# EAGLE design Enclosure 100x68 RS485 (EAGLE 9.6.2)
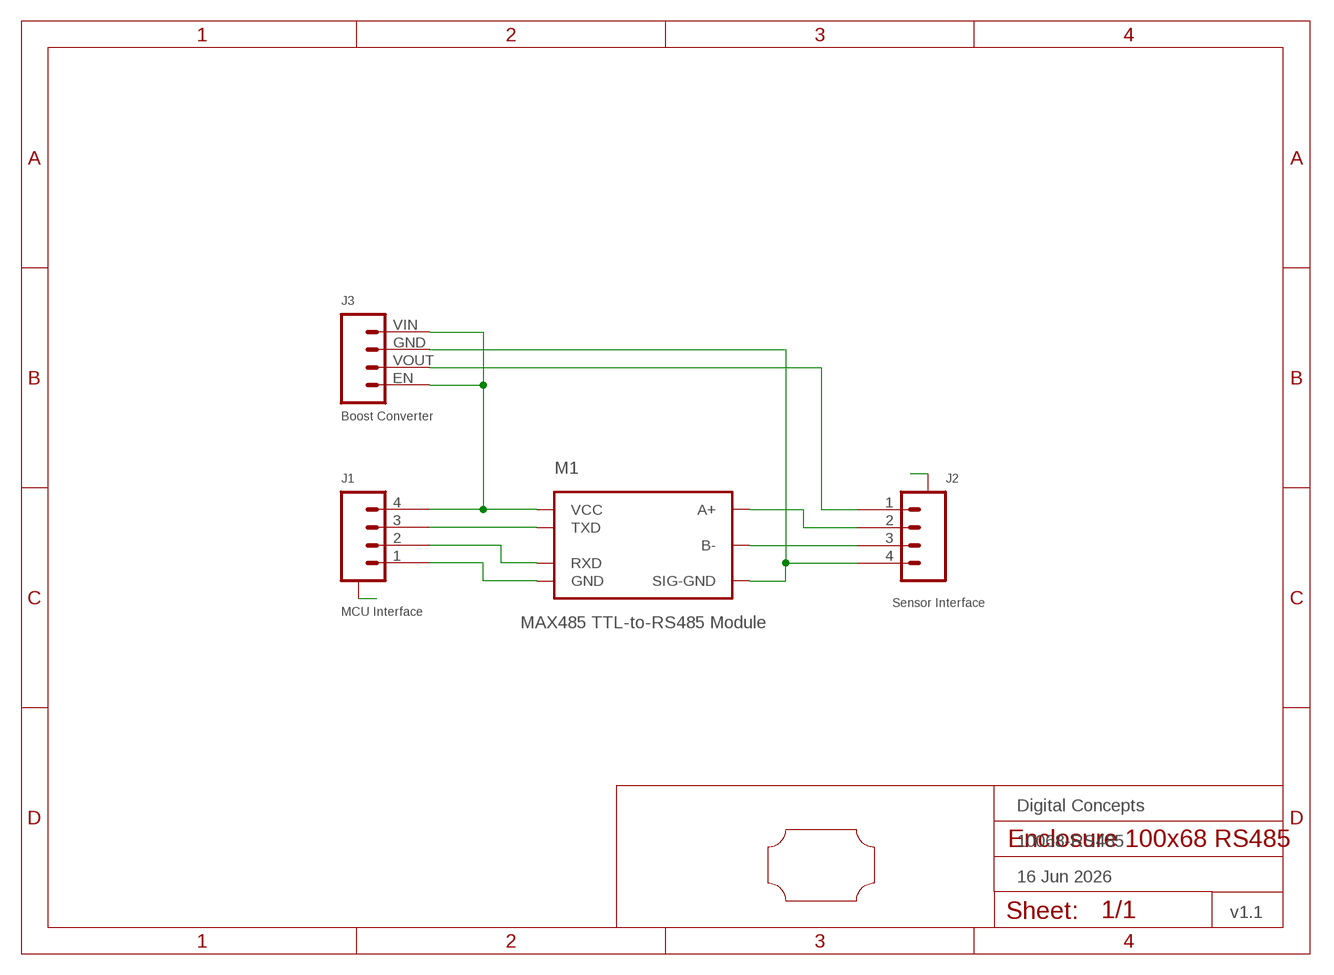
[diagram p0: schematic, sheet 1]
FRAME1 (FRAME_A5L-LOC): DATE: 16 Jun 2026; OWNER: Digital Concepts; TITLE: 10068-RS485; VERSION: v1.1

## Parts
J1  MCU Interface  JST-SH1.0-4-SMD-HORIZONTAL  [JST-SH1.0-4-SMD-HORIZONTAL]
J2  Sensor Interface  JST-SH1.0-4-SMD-HORIZONTAL  [JST-SH1.0-4-SMD-HORIZONTAL]
J3  Boost Converter  HEADER-1X4-BOOST  [CONN_04-BOOST]
M1  MAX485 TTL-to-RS485 Module  MAX485-MODULE  [MAX485-MODULE]
U$1  PROTO-34X22-RS485  [PROTO-34X22-RS485]

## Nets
A1: J2.A@1(A) J2.A@4(A)
A2: J1.A@1(A) J1.A@4(A)
A+: J2.2 M1.A+
B-: J2.3 M1.B-
GND: J1.1 M1.GND
RXD: J1.2 M1.RXD
SIG-GND: J2.4 J3.GND M1.SIG-GND
TXD: J1.3 M1.TXD
VCC: J1.4 J3.EN J3.VIN M1.VCC
VDD: J2.1 J3.VOUT

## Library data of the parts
J1 J2 = digitalconcepts:JST-SH1.0-4-SMD-HORIZONTAL: JST SH1.0 4P SMD horizontal connector
J3 = digitalconcepts:HEADER-1X4-BOOST: Boost Converter Module 4-Pin Header
M1 = digitalconcepts:MAX485-MODULE: MAX485 TTL-to-RS485 Adaptor Module
U$1 = digitalconcepts:PROTO-34X22-RS485: 34 x 22 Prototyping board, with cut-outs, to fit an 100 x 68 enclosure

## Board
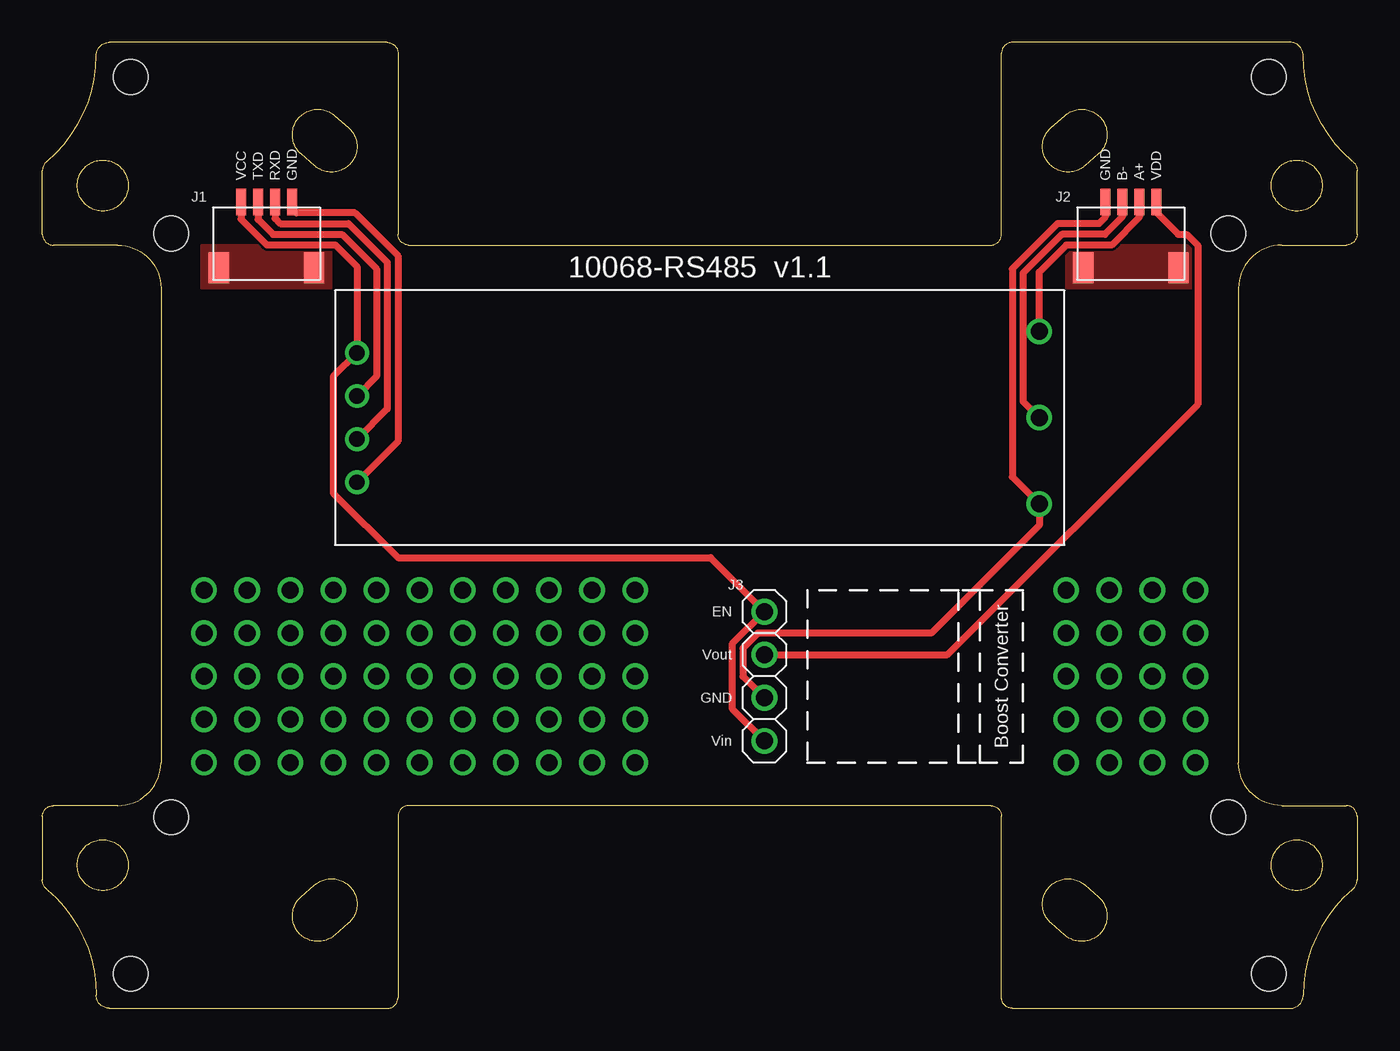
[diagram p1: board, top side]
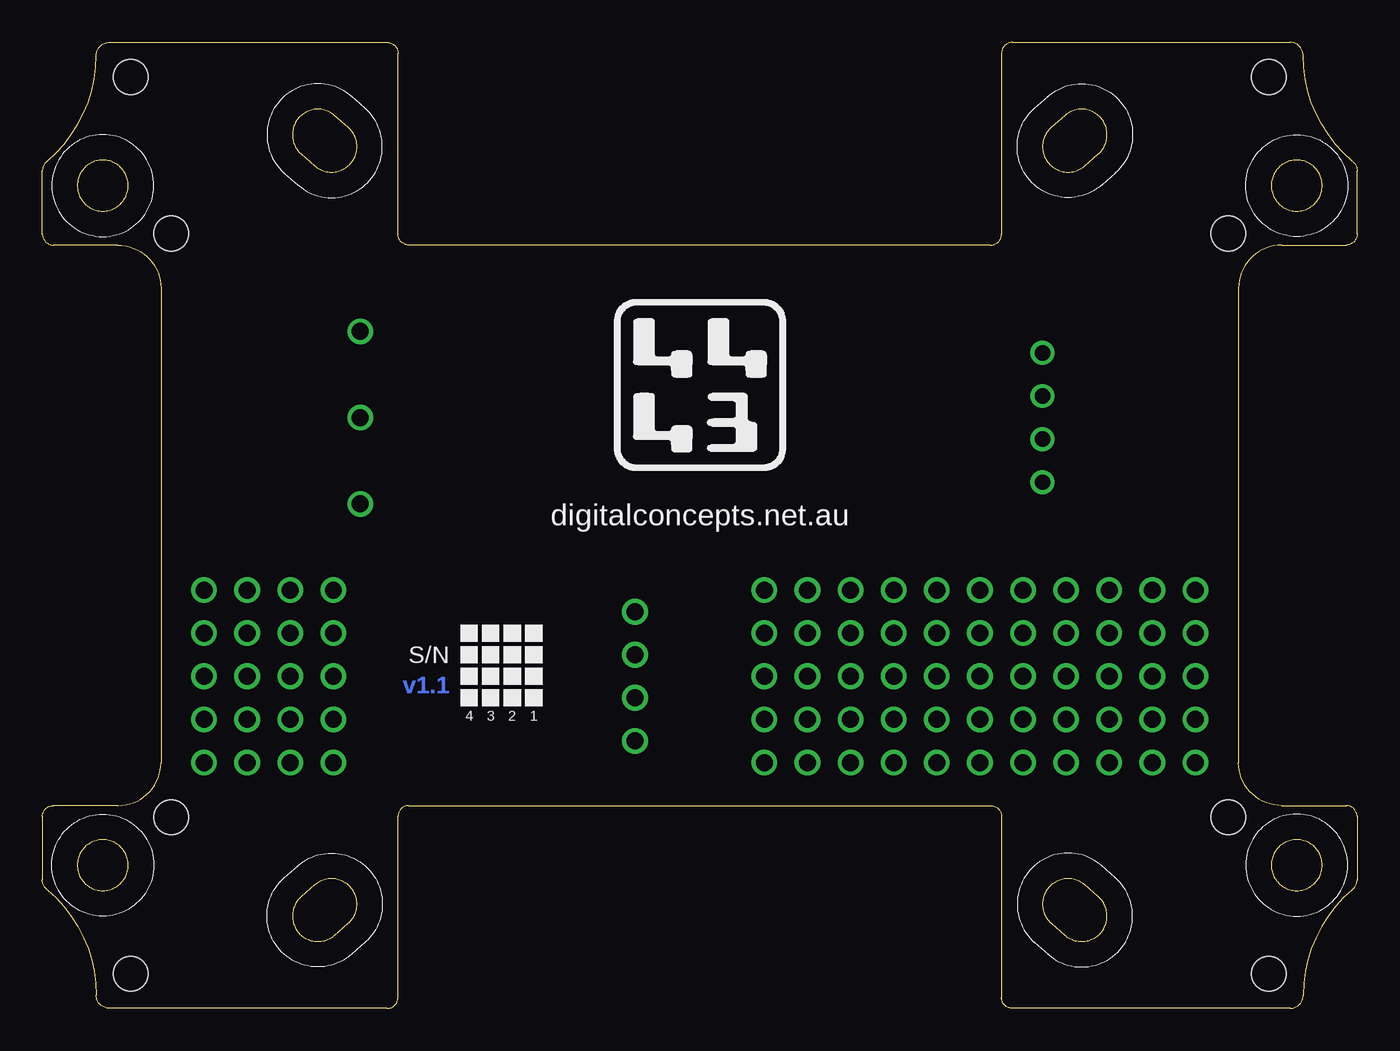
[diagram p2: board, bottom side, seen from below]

Size 77.47 x 56.9 mm. Coordinates in mm from the lower left corner, seen from the top.
Copper layers (1*16): Top 0.035mm / dielectric 1.5mm / Bottom 0.035mm
Design rules "default *": minimum track width 6mil, minimum drill 0.35mm, track to track 6mil, track to pad 6mil, pad to pad 6mil, via to via 6mil, smd to smd 6mil, copper to edge 6mil, drill to drill 6mil, minimum pad ring 10mil, minimum via ring 8mil, stop-mask expansion 4mil, vias tented up to drill 0mil, thermal gap 10mil

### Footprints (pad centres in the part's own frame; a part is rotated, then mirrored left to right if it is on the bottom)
JST-SH1.0-4-SMD-HORIZONTAL = smd 0.6 x 1.55: 1 1.5,2.54; 2 0.5,2.54; 3 -0.5,2.54; 4 -1.5,2.54 | smd 1.2 x 1.8: A@1 2.8,-1.335; A@4 -2.8,-1.335
CONN_04-BOOST = drill 1 pad 1.524: EN 0,0; GND 5.08,0; VIN 7.62,0; VOUT 2.54,0
MAX485-MODULE = drill 1: A+ 20,5.08; B- 20,0; SIG-GND 20,-5.08 | drill 0.9: GND -20.2,-3.81; RXD -20.2,-1.27; TXD -20.2,1.27; VCC -20.2,3.81
PROTO-34X22-RS485 = drill 1: P06-06 -29.21,-13.97; P06-07 -29.21,-11.43; P06-08 -29.21,-8.89; P06-09 -29.21,-6.35; P06-10 -29.21,-3.81; P07-06 -26.67,-13.97; P07-07 -26.67,-11.43; P07-08 -26.67,-8.89; P07-09 -26.67,-6.35; P07-10 -26.67,-3.81; P08-06 -24.13,-13.97; P08-07 -24.13,-11.43; P08-08 -24.13,-8.89; P08-09 -24.13,-6.35; P08-10 -24.13,-3.81; P09-06 -21.59,-13.97; P09-07 -21.59,-11.43; P09-08 -21.59,-8.89; P09-09 -21.59,-6.35; P09-10 -21.59,-3.81; P10-06 -19.05,-13.97; P10-07 -19.05,-11.43; P10-08 -19.05,-8.89; P10-09 -19.05,-6.35; P10-10 -19.05,-3.81; P11-06 -16.51,-13.97; P11-07 -16.51,-11.43; P11-08 -16.51,-8.89; P11-09 -16.51,-6.35; P11-10 -16.51,-3.81; P12-06 -13.97,-13.97; P12-07 -13.97,-11.43; P12-08 -13.97,-8.89; P12-09 -13.97,-6.35; P12-10 -13.97,-3.81; P13-06 -11.43,-13.97; P13-07 -11.43,-11.43; P13-08 -11.43,-8.89; P13-09 -11.43,-6.35; P13-10 -11.43,-3.81; P14-06 -8.89,-13.97; P14-07 -8.89,-11.43; P14-08 -8.89,-8.89; P14-09 -8.89,-6.35; P14-10 -8.89,-3.81; P15-06 -6.35,-13.97; P15-07 -6.35,-11.43; P15-08 -6.35,-8.89; P15-09 -6.35,-6.35; P15-10 -6.35,-3.81; P16-06 -3.81,-13.97; P16-07 -3.81,-11.43; P16-08 -3.81,-8.89; P16-09 -3.81,-6.35; P16-10 -3.81,-3.81; P26-06 21.59,-13.97; P26-07 21.59,-11.43; P26-08 21.59,-8.89; P26-09 21.59,-6.35; P26-10 21.59,-3.81; P27-06 24.13,-13.97; P27-07 24.13,-11.43; P27-08 24.13,-8.89; P27-09 24.13,-6.35; P27-10 24.13,-3.81; P28-06 26.67,-13.97; P28-07 26.67,-11.43; P28-08 26.67,-8.89; P28-09 26.67,-6.35; P28-10 26.67,-3.81; P29-06 29.21,-13.97; P29-07 29.21,-11.43; P29-08 29.21,-8.89; P29-09 29.21,-6.35; P29-10 29.21,-3.81 | hole 2.032: -33.528,26.416; 33.528,26.416; 33.528,-26.416; -33.528,-26.416; -31.14,17.196; 31.14,17.196; -31.14,-17.196; 31.14,-17.196

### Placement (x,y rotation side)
J1  13.21,44.96 0 top
J2  64.14,44.96 0 top
J3  42.55,23.37 270 top
M1  38.73,34.8 0 top
U$1  38.73,28.45 0 top

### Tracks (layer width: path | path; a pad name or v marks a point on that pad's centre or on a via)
A1
  pour Top (no thermals): 60.33,42.42 67.94,42.42 67.94,44.96 60.33,44.96
A2
  pour Top (no thermals): 9.4,44.96 17.02,44.96 17.02,42.42 9.4,42.42
A+
  Top 0.406: J2.2 64.64,46.59 63.01,44.96 60.33,44.96 58.73,43.37 M1.A+
B-
  Top 0.406: M1.B- 57.78,35.75 57.78,43.31 60.07,45.59 62.61,45.59 63.64,46.62 J2.3
GND
  Top 0.406: J1.1 14.71,47.12 14.96,46.86 18.41,46.86 20.95,44.32 20.95,33.41 M1.GND
RXD
  Top 0.406: J1.2 13.71,46.54 14.02,46.23 18.03,46.23 20.32,43.94 20.32,35.31 M1.RXD
SIG-GND
  Top 0.406: J2.4 62.64,46.61 62.25,46.23 59.82,46.23 57.15,43.56 57.15,31.3 M1.SIG-GND 58.73,28.45 52.38,22.1 42.16,22.1 41.27,21.21 41.27,19.56 J3.GND
TXD
  Top 0.406: J1.3 12.71,46.47 13.59,45.59 17.65,45.59 19.68,43.56 19.68,37.22 M1.TXD
VCC
  Top 0.406: J1.4 11.71,46.48 13.23,44.96 17.26,44.96 18.53,43.69 M1.VCC 17.14,37.22 17.14,30.35 20.95,26.54 39.37,26.54 J3.EN 40.64,21.46 40.64,17.65 J3.VIN
VDD
  Top 0.406: J2.1 65.64,46.89 66.93,45.59 67.44,45.59 68.07,44.96 68.07,35.56 53.34,20.83 J3.VOUT

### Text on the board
Bottom: v1.1
tPlace: 10068-RS485 v1.1
bPlace: digitalconcepts.net.au | S/N | 1 | 2 | 3 | 4
tNames: VCC | TXD | RXD | GND | GND | B- | A+ | VDD | EN | Vout | GND | Vin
